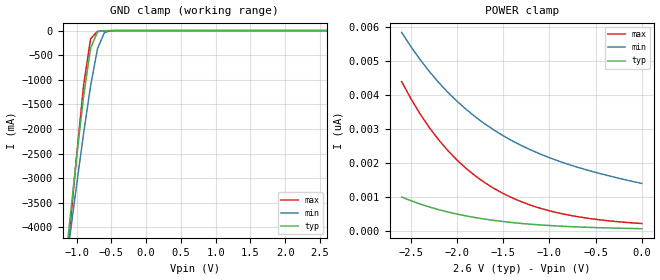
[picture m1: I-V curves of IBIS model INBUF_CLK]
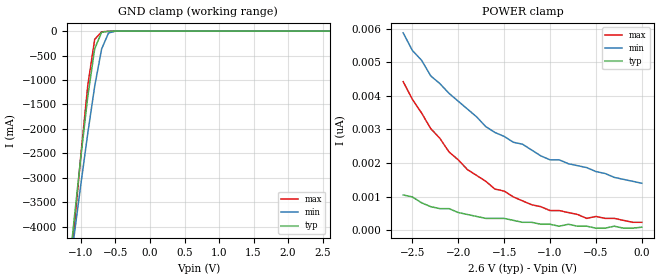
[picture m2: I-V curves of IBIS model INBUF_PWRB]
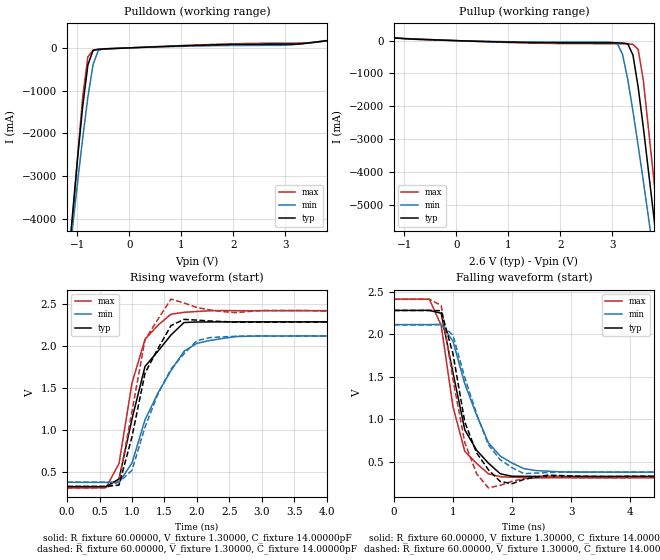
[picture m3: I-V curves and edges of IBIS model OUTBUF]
| IBIS file cspt857_tssop_3200.ibs created by s2ibis2 version 1.2
| North Carolina State University Electronics Research Laboratory  1995
[IBIS ver]   2.1
[File name]   cspt857_tssop_3200.ibs
[File Rev]   1.0
[Date]   Monday, August 25, 2003
[Source]   IDT
[Notes]   1. Temp typ=25C, min=0C, max=100C
   2. IDT's 2.0v C11.5 process
   3. Ramp rate based on 50 ohm load
READ THESE TERMS AND CONDITIONS CAREFULLY BEFORE USING THIS IBIS MODEL.  BY
USING THIS IBIS MODEL, YOU ARE ACCEPTING AND AGREEING TO THESE TERMS AND
CONDITIONS OF USE.
Integrated Device Technology, Inc. ("IDT") hereby grants the user of this
IBIS model ("User") a non-exclusive, nontransferable license to use this
IBIS model under the following terms: The User is granted this license only
to use the IBIS model for demonstration purposes only and is not granted
rights to sell, copy (except as needed to run the IBIS model), rent, lease
or sub-license (except for demonstration) the IBIS model in whole or in
part, or in modified form to anyone. The User may modify the IBIS model to
suit its specific applications, but  rights to derivative works and such
modifications shall belong to IDT.
THIS IBIS MODEL IS PROVIDED ON AN AS IS" BASIS AND IDT  MAKES ABSOLUTELY NO
WARRANTY WITH RESPECT TO THE INFORMATION CONTAINED HEREIN.  IDT DISCLAIMS
AND USER WAIVES ALL WARRANTIES, EXPRESS AND IMPLIED, INCLUDING WARRANTIES OF
MERCHANTABILITY AND FITNESS FOR A PARTICULAR PURPOSE.  THE ENTIRE RISK AS TO
QUALITY AND PERFORMANCE IS WITH THE USER  ACCORDINGLY, IN NO EVENT SHALL IDT
BE LIABLE FOR ANY DIRECT OR INDIRECT DAMAGES, WHETHER IN CONTRACT OR TORT,
INCLUDING ANY LOST PROFITS OR OTHER INCIDENTAL, CONSEQUENTIAL, EXEMPLARY, OR
PUNITIVE DAMAGES ARISING OUT OF THE USE OR APPLICATION OF THE  IBIS MODEL,
WHETHER OR NOT IDT HAD NOTICE OF SUCH DAMAGES.
IDT reserves the right to make changes without notice to any product herein
to improve
reliability, function, or design. IDT does not convey any license under
patent rights or any other intellectual property rights, including those of
third parties. IDT is not obligated
to provide maintenance or support for the licensed IBIS model.
This model is for the 2.5V Phase Locked Loop Differential 1:10 SDRAM Clock
Driver
[Copyright]
Copyright 2002, Integrated Device Technology, Inc. All rights reserved.
|   Component CPST857C
[Component]   CPST857C
[Manufacturer]   Integrated Device Technology Inc.
[Package]
|Following package parameters are for TSSOP 48 lead packa
| variable   typ   min   max
R_pkg   0.10400   77.000000m   0.13000
L_pkg   3.20000nH   2.50000nH   4.40000nH
C_pkg   0.27000pF   0.17000pF   0.39000pF
[Pin]  signal_name   model_name   R_pin   L_pin   C_pin
1   GND   GND
2   _Y0_   OUTBUF
3   Y0   OUTBUF
4   VDDQ   POWER
5   Y1   OUTBUF
6   _Y1_   OUTBUF
7   GND   GND
8   GND   GND
9   _Y2_   OUTBUF
10   Y2   OUTBUF
11   VDDQ   POWER
12   VDDQ   POWER
13   CLK   INBUF_CLK
14   _CLK_   INBUF_CLK
15   VDDQ   POWER
16   AVDD   POWER
17   AGND   GND
18   GND   GND
19   _Y3_   OUTBUF
20   Y3   OUTBUF
21   VDDQ   POWER
22   Y4   OUTBUF
23   _Y4_   OUTBUF
24   GND   GND
25   GND   GND
26   _Y9_   OUTBUF
27   Y9   OUTBUF
28   VDDQ   POWER
29   Y8   OUTBUF
30   _Y8_   OUTBUF
31   GND   GND
32   FBOUT   OUTBUF
33   _FBOUT_   OUTBUF
34   VDDQ   POWER
35   _FBIN_   INBUF_FBIN
36   FBIN   INBUF_FBIN
37   _PWRDWN_   INBUF_PWRB
38   VDDQ   POWER
39   Y7   OUTBUF
40   _Y7_   OUTBUF
41   GND   GND
42   GND   GND
43   _Y6_   OUTBUF
44   Y6   OUTBUF
45   VDDQ   POWER
46   Y5   OUTBUF
47   _Y5_   OUTBUF
48   GND   GND
| in   in   dummy_model
| *oe  oe   dummy_model
[Diff Pin]  inv_pin  vdiff   tdelay_typ  tdelay_min  tdelay_max
13   14   1.00V   NA   |CLK<P:N> Clock Input pair
36   35   1.00V   NA   |FBIN<P:N> FBIN Input pair
3   2   0.000V   NA   |YX<P:N> Output pair
5   6   0.000V   NA   |YX<P:N> Output pair
10   9   0.000V   NA   |YX<P:N> Output pair
20   19   0.000V   NA   |YX<P:N> Output pair
22   23   0.000V   NA   |YX<P:N> Output pair
27   26   0.000V   NA   |YX<P:N> Output pair
29   30   0.000V   NA   |YX<P:N> Output pair
32   33   0.000V   NA   |YX<P:N> Output pair
39   40   0.000V   NA   |YX<P:N> Output pair
44   43   0.000V   NA   |YX<P:N> Output pair
46   47   0.000V   NA   |YX<P:N> Output pair
[Pin Mapping]  pulldown_ref   pullup_ref   gnd_clamp_ref  power_clamp_ref
1   GND   NC
2   GND   VDDQ
3   GND   VDDQ
4   NC   VDDQ
5   GND   VDDQ
6   GND   VDDQ
7   GND   NC
8   GND   NC
9   GND   VDDQ
10   GND   VDDQ
11   NC   VDDQ
12   NC   VDDQ
13   NC   NC   GND   VDDQ
14   NC   NC   GND   VDDQ
15   NC   VDDQ
16   NC   AVDD
17   AGND   NC
18   GND   NC
19   GND   VDDQ
20   GND   VDDQ
21   NC   VDDQ
22   GND   VDDQ
23   GND   VDDQ
24   GND   NC
25   GND   NC
26   GND   VDDQ
27   GND   VDDQ
28   NC   VDDQ
29   GND   VDDQ
30   GND   VDDQ
31   GND   NC
32   GND   VDDQ
33   GND   VDDQ
34   NC   VDDQ
35   NC   NC   GND   VDDQ
36   NC   NC   GND   VDDQ
37   NC   NC   GND   VDDQ
38   NC   VDDQ
39   GND   VDDQ
40   GND   VDDQ
41   GND   NC
42   GND   NC
43   GND   VDDQ
44   GND   VDDQ
45   NC   VDDQ
46   GND   VDDQ
47   GND   VDDQ
48   GND   NC
| Models and submodels in the file (4): INBUF_CLK (Input), INBUF_PWRB (Input), INBUF_FBIN (Input), OUTBUF (Output)
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|   Model INBUF_CLK
[Model]   INBUF_CLK
Model_type   Input
Polarity   Non-Inverting
Vinl =  0.80000V
Vinh =  2.00000V
C_comp   2.30000pF   2.30000pF   2.30000pF
[Temperature Range]   25.00000   100.00000   0.000
[Voltage Range]   2.60000V   2.50000V   2.70000V
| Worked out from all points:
|   GND clamp passes 1 mA (typ) near -0.52 V on its own axis
[GND_clamp]
| voltage   I(typ)   I(min)   I(max)
-2.6V     -25.34A    -21.53A    -29.72A
-1.2V     -5.248A    -5.316A    -5.713A
-1.1V     -3.884A    -4.209A    -4.089A
-1V       -2.564A    -3.127A    -2.526A
-900mV    -1.335A    -2.086A    -1.108A
-800mV    -361.3mA   -1.127A    -168.2mA
-700mV    -23.9mA    -365.3mA   -14.69mA
-600mV    -2.784mA   -39.09mA   -5.291mA
-500mV    -459.2uA   -2.159mA   -1.358mA
2.6V      75.77pA    1.461nA    209.7pA
[POWER_clamp]
| voltage   I(typ)   I(min)   I(max)
-2.6V     1.003nA    5.831nA    4.388nA
-2.5V     895.5pA    5.414nA    3.887nA
-2.4V     798.8pA    5.033nA    3.439nA
-2.3V     712pA      4.684nA    3.039nA
-2.1V     565pA      4.076nA    2.367nA
-1.9V     448.2pA    3.57nA     1.838nA
-1.8V     399.3pA    3.35nA     1.618nA
-1.6V     317.8pA    2.967nA    1.255nA
-1.3V     228.2pA    2.509nA    861.2pA
-900mV    152.1pA    2.058nA    534.7pA
-500mV    107.5pA    1.726nA    349.9pA
0V        75.77pA    1.402nA    226.3pA
|   Model INBUF_PWRB
[Model]   INBUF_PWRB
Model_type   Input
Polarity   Non-Inverting
Vinl =  0.80000V
Vinh =  2.00000V
C_comp   2.30000pF   2.30000pF   2.30000pF
[Temperature Range]   25.00000   100.00000   0.000
[Voltage Range]   2.60000V   2.50000V   2.70000V
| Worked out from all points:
|   GND clamp passes 1 mA (typ) near -0.52 V on its own axis
[GND_clamp]
| voltage   I(typ)   I(min)   I(max)
-2.6V     -25.34A    -21.53A    -29.72A
-1.2V     -5.247A    -5.316A    -5.712A
-1.1V     -3.884A    -4.209A    -4.088A
-1V       -2.564A    -3.127A    -2.526A
-900mV    -1.335A    -2.086A    -1.108A
-800mV    -361.3mA   -1.126A    -168.2mA
-700mV    -23.9mA    -365.3mA   -14.69mA
-600mV    -2.784mA   -39.09mA   -5.291mA
-500mV    -459.2uA   -2.159mA   -1.358mA
2.6V      87.31pA    1.455nA    232.8pA
[POWER_clamp]
| voltage   I(typ)   I(min)   I(max)
-2.6V     1.048nA    5.879nA    4.424nA
-2.5V     989.5pA    5.355nA    3.9nA
-2.4V     814.9pA    5.064nA    3.492nA
-2.3V     698.5pA    4.598nA    3.027nA
-2.2V     640.3pA    4.366nA    2.736nA
-2.1V     640.3pA    4.075nA    2.328nA
-1.9V     465.7pA    3.609nA    1.804nA
-1.6V     349.2pA    2.91nA     1.222nA
-1V       174.6pA    2.095nA    582.1pA
-600mV    116.4pA    1.863nA    349.2pA
-500mV    58.21pA    1.746nA    407.5pA
0V        87.31pA    1.397nA    232.8pA
|   Model OUTBUF
[Model]   OUTBUF
Model_type   Output
Polarity   Non-Inverting
Vmeas =  1.30000V
C_comp   4.80000pF   4.80000pF   4.80000pF
[Temperature Range]   25.00000   100.00000   0.000
[Voltage Range]   2.60000V   2.50000V   2.70000V
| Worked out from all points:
|   slope of the pulldown table from 0 to 0.39 V, typ, clamps not added: 20.1 ohm
|   slope of the pullup table from 0 to 0.39 V, typ, clamps not added: 19.5 ohm
|   rising waveform, R_fixture 60.00000, V_fixture 1.30000, C_fixture 14.00000pF: 20-80 % time 468ps typ, 610ps min, 341ps max; typ from 0.326 V to 2.28 V
|   rising waveform, R_fixture 60.00000, V_fixture 1.30000, C_fixture 14.00000pF: 20-80 % time 418ps typ, 570ps min, 299ps max; typ from 0.327 V to 2.28 V
|   falling waveform, R_fixture 60.00000, V_fixture 1.30000, C_fixture 14.00000pF: 20-80 % time 429ps typ, 539ps min, 335ps max; typ from 2.28 V to 0.326 V
|   falling waveform, R_fixture 60.00000, V_fixture 1.30000, C_fixture 14.00000pF: 20-80 % time 384ps typ, 496ps min, 318ps max; typ from 2.28 V to 0.327 V
[Pulldown]
| voltage   I(typ)   I(min)   I(max)
-2.6V     -25.48A    -21.66A    -29.86A
-1.2V     -5.305A    -5.362A    -5.777A
-1V       -2.612A    -3.165A    -2.58A
-900mV    -1.379A    -2.12A     -1.157A
-800mV    -400.6mA   -1.157A    -211.8mA
-700mV    -58.58mA   -392.6mA   -53.12mA
-600mV    -32.75mA   -62.73mA   -38.49mA
-500mV    -25.6mA    -22.07mA   -29.24mA
1.8V      74.65mA    53.14mA    87.89mA
3V        87.07mA    61.25mA    109.7mA
3.3V      95.16mA    92.97mA    112.3mA
5.2V      400.4mA    370.7mA    414.1mA
[Pullup]
| voltage   I(typ)   I(min)   I(max)
-2.6V     302.8mA    288.1mA    310.8mA
-900mV    51.47mA    51.29mA    59.76mA
1.3V      -54.7mA    -38.46mA   -68.74mA
3.1V      -70.01mA   -89.45mA   -94.24mA
3.2V      -73.17mA   -420.6mA   -95.98mA
3.3V      -96.9mA    -1.187A    -101.2mA
3.4V      -439.3mA   -2.153A    -112.7mA
3.5V      -1.419A    -3.2A      -270mA
3.6V      -2.655A    -4.288A    -1.216A
3.8V      -5.352A    -6.531A    -4.21A
4V        -8.161A    -8.821A    -7.507A
5.2V      -25.55A    -22.89A    -28.21A
[Ramp]
| variable   typ   min   max
dV/dt_r   1.09920/0.10519n   0.93300/0.15232n   1.21080/0.13672n
dV/dt_f   1.10088/0.14109n   0.96540/0.13417n   1.18398/0.13634n
R_load = 50.00000
[Rising Waveform]
R_fixture = 60.00000
V_fixture = 1.30000
V_fixture_min = 1.25000
V_fixture_max = 1.35000
C_fixture = 14.00000pF
| time   V(typ)   V(min)   V(max)
0s        325.5mV    375.9mV    310.2mV
600ps     325.4mV    375.9mV    313.6mV
800ps     415.9mV    374.8mV    599.6mV
1ns       1.132V     607mV      1.557V
1.2ns     1.754V     1.119V     2.076V
1.6ns     2.128V     1.704V     2.376V
1.8ns     2.276V     1.935V     2.397V
2ns       2.283V     2.029V     2.408V
2.6ns     2.284V     2.109V     2.417V
10ns      2.284V     2.116V     2.417V
[Rising Waveform]
R_fixture = 60.00000
V_fixture = 1.30000
V_fixture_min = 1.25000
V_fixture_max = 1.35000
C_fixture = 14.00000pF
R_dut = 0.10400
L_dut = 3.20000nH
C_dut = 0.27000pF
| time   V(typ)   V(min)   V(max)
0s        326.8mV    377mV      311.6mV
600ps     326.7mV    377mV      311.7mV
800ps     343.6mV    376.5mV    387mV
1ns       920.1mV    520.6mV    1.224V
1.2ns     1.674V     1.033V     2.071V
1.4ns     1.968V     1.428V     2.317V
1.6ns     2.24V      1.722V     2.554V
2ns       2.305V     2.061V     2.454V
2.2ns     2.295V     2.097V     2.426V
10ns      2.283V     2.115V     2.415V
[Falling Waveform]
R_fixture = 60.00000
V_fixture = 1.30000
V_fixture_min = 1.25000
V_fixture_max = 1.35000
C_fixture = 14.00000pF
| time   V(typ)   V(min)   V(max)
0s        2.284V     2.116V     2.417V
600ps     2.285V     2.116V     2.415V
800ps     2.25V      2.12V      2.108V
1ns       1.547V     1.92V      1.147V
1.2ns     874.7mV    1.418V     621.2mV
1.4ns     634.4mV    1.047V     478.8mV
1.6ns     482.4mV    723.4mV    356.9mV
1.8ns     356.9mV    565.6mV    322.2mV
2.4ns     326mV      395.1mV    309.7mV
10ns      325.5mV    375.9mV    310.2mV
[Falling Waveform]
R_fixture = 60.00000
V_fixture = 1.30000
V_fixture_min = 1.25000
V_fixture_max = 1.35000
C_fixture = 14.00000pF
R_dut = 0.10400
L_dut = 3.20000nH
C_dut = 0.27000pF
| time   V(typ)   V(min)   V(max)
0s        2.283V     2.115V     2.415V
600ps     2.283V     2.115V     2.415V
800ps     2.281V     2.116V     2.343V
1ns       1.771V     1.991V     1.47V
1.2ns     966.3mV    1.491V     724.1mV
1.4ns     603.2mV    1.063V     357.2mV
1.6ns     403.8mV    697.5mV    190.6mV
1.8ns     265.8mV    522.2mV    220.7mV
2.2ns     290.5mV    358.3mV    300.4mV
10ns      326.8mV    377mV      311.6mV
